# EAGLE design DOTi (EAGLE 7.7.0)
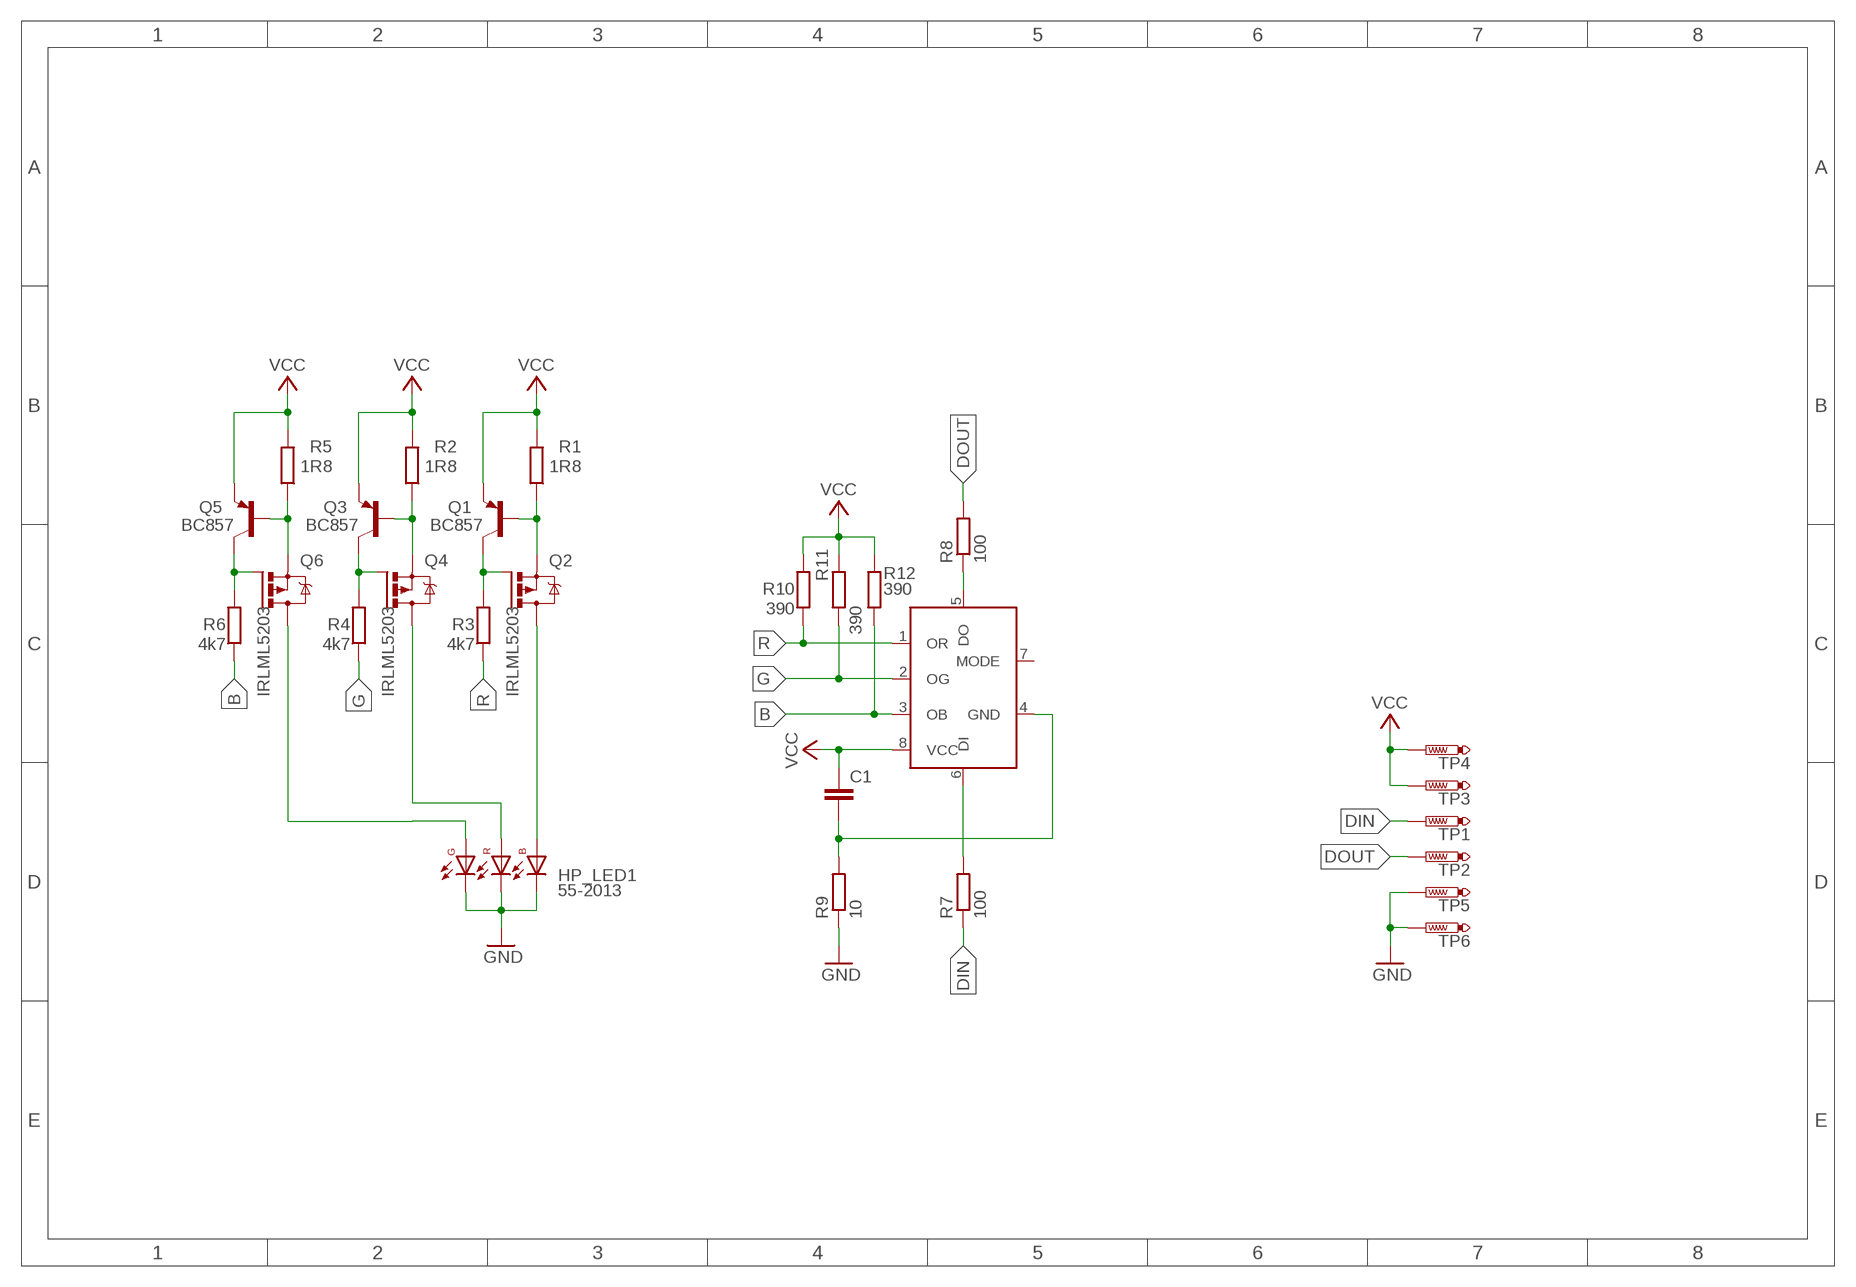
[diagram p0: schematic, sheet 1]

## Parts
C1  C-EUC0603  [C0603]
HP_LED1  55-2013  [HP_RGB_LED]
IC1  WS2811M  [MSOP8]
Q1  BC857  BC857CSMD  [SOT23-BEC]
Q2  IRLML5203  [MICRO3]
Q3  BC857  BC857CSMD  [SOT23-BEC]
Q4  IRLML5203  [MICRO3]
Q5  BC857  BC857CSMD  [SOT23-BEC]
Q6  IRLML5203  [MICRO3]
R1  1R8  R-EU_M1206  [M1206]
R2  1R8  R-EU_M1206  [M1206]
R3  4k7  R-EU_R0603  [R0603]
R4  4k7  R-EU_R0603  [R0603]
R5  1R8  R-EU_M1206  [M1206]
R6  4k7  R-EU_R0603  [R0603]
R7  100  R-EU_R0603  [R0603]
R8  100  R-EU_R0603  [R0603]
R9  10  R-EU_R0603  [R0603]
R10  390  R-EU_R0603  [R0603]
R11  390  R-EU_R0603  [R0603]
R12  390  R-EU_R0603  [R0603]
TP1  PTR1B1,27  [B1,27]
TP2  PTR1B1,27  [B1,27]
TP3  PTR1B1,27  [B1,27]
TP4  PTR1B1,27  [B1,27]
TP5  PTR1B1,27  [B1,27]
TP6  PTR1B1,27  [B1,27]

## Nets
B: IC1.3(OB) R6.1 R12.1
DI: IC1.6(DI) R7.2
DIN: R7.1 TP1.TP
DO: IC1.5(DO) R8.1
DOUT: R8.2 TP2.TP
G: IC1.2(OG) R4.1 R11.1
GND: HP_LED1.1(GC) HP_LED1.2(RC) HP_LED1.3(BC) R9.1 TP5.TP TP6.TP
N$1: HP_LED1.5(RA) Q4.3(D)
N$2: Q1.B Q2.2(S) R1.1
N$3: Q1.C Q2.1(G) R3.2
N$4: HP_LED1.4(BA) Q2.3(D)
N$5: HP_LED1.6(GA) Q6.3(D)
N$6: Q3.B Q4.2(S) R2.1
N$7: Q5.B Q6.2(S) R5.1
N$9: Q3.C Q4.1(G) R4.2
N$11: Q5.C Q6.1(G) R6.2
N$12: C1.2 IC1.4(GND) R9.2
R: IC1.1(OR) R3.1 R10.1
VCC: C1.1 IC1.8(VCC) Q1.E Q3.E Q5.E R1.2 R2.2 R5.2 R10.2 R11.2 R12.2 TP3.TP TP4.TP
Unconnected: IC1.7(MODE)

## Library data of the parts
C1 = rcl:C-EU: CAPACITOR, European symbol
HP_LED1 = RGB_HP_LED:55-2013
IC1 = WS2812:WS2811M
Q1 Q3 Q5 = transistor-pnp:BC857*: PNP Transistror
Q2 Q4 Q6 = transistor-power:IRLML5203: HEXFET P-Channel Power MOSFET
R1-R12 = rcl:R-EU_: RESISTOR, European symbol
TP1-TP6 = testpad:PTR1: TEST PIN

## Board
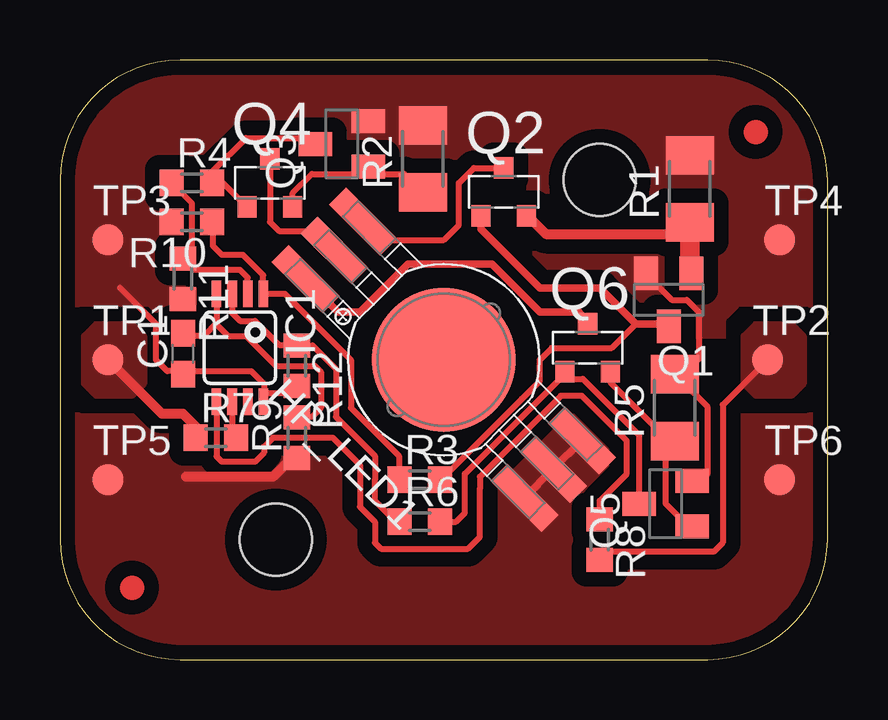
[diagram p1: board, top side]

Size 32 x 25 mm. Coordinates in mm from the lower left corner, seen from the top.
Outline: 5,0 27,0 arc90 32,5 32,20 arc90 27,25 5,25 arc90 0,20 0,5 arc90 5,0
Copper layers (1*16): Top 0.035mm / dielectric 1.5mm / Bottom 0.035mm
Design rules "default *": minimum track width 10mil, minimum drill 24mil, track to track 8mil, track to pad 8mil, pad to pad 8mil, via to via 8mil, smd to smd 8mil, copper to edge 20mil, drill to drill 8mil, minimum pad ring 10mil, minimum via ring 8mil, stop-mask expansion 4mil, vias tented up to drill 0mil, thermal gap 10mil
Holes 3 mm at 9,5 22.5,20

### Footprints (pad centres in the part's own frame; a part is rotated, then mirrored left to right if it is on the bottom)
C0603 = smd 1.1 x 1: 1 -0.85,0; 2 0.85,0
HP_RGB_LED = smd 3 x 1: 1 -6.45,1.7; 2 -6.45,0; 3 -6.45,-1.7; 4 6.45,-1.7; 5 6.45,0; 6 6.45,1.7 | smd 6 x 6: P$1 0,0
MSOP8 = smd 1.1 x 0.4: 1 -2.25,0.975; 2 -2.25,0.325; 3 -2.25,-0.325; 4 -2.25,-0.975; 5 2.25,-0.975; 6 2.25,-0.325; 7 2.25,0.325; 8 2.25,0.975
SOT23-BEC = smd 1 x 1.4: B -0.95,-1.1; C 0,1.1; E 0.95,-1.1
MICRO3 = smd 0.8 x 0.9: 1 -0.95,-1; 2 0.95,-1; 3 0,1
M1206 = smd 1.6 x 2: 1 -1.4,0; 2 1.4,0
R0603 = smd 1 x 1.1: 1 -0.85,0; 2 0.85,0
B1,27 = smd 1.27 x 1.27: TP 0,0

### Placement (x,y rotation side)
C1  5.12,12.75 90 top
HP_LED1  16,12.5 135 top
IC1  7.5,13 270 top
Q1  25.38,15 180 top
Q2  18.5,19.5 0 top
Q3  11.75,21.5 90 top
Q4  8.75,19.88 0 top
Q5  25.25,6.5 90 top
Q6  22,13 0 top
R1  26.25,19.62 90 top
R2  15.12,20.88 90 top
R3  15,7.5 0 top
R4  5.5,19.88 0 top
R5  25.62,10.5 90 top
R6  15,5.75 0 top
R7  6.5,9.25 0 top
R8  22.5,5 270 top
R9  9.88,9.25 90 top
R10  5.5,18.25 180 top
R11  5.12,15.88 270 top
R12  9.88,12.25 270 top
TP1  2,12.5 0 top
TP2  29.5,12.5 0 top
TP3  2,17.5 0 top
TP4  30,17.5 0 top
TP5  2,7.5 0 top
TP6  30,7.5 0 top

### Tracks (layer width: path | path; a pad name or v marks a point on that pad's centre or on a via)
B
  Top 0.254: IC1.3 7.17,14.45 7.5,14.12 8.12,14.12 9.12,13.12 9.85,13.12 R12.1 10.53,13.1 11.25,12.38 11.5,12.12 11.5,10.12 13.12,8.5 13.12,7.5 13.12,6.62 14,5.75
  Top 0.305: R6.1 14,5.75
DI
  Top 0.254: IC1.6 7.17,9.3 R7.2
DIN
  Top 0.254: 2.5,12 TP1.TP
  Top 0.406: R7.1 5.65,9.72 5.12,10.25 4.25,10.25 3.62,10.88 2.5,12
  pour Top (no thermals): 1,11.5 1,13.5 1.5,14 3,14 3.5,13.5 3.5,11.5 3,11 1.5,11
DO
  Top 0.254: R8.1 22.5,6.62 23.62,7.75 23.62,9.12 23.25,9.5 21.75,11 20.88,11 17.5,7.62 17.5,7.12 17.5,5.12 17,4.62 13.38,4.62 13.12,4.88 13.12,5.75 12.5,6.38 12.5,8.12 11.75,8.88 11.38,9.25 8.88,9.25 8.5,8.88 8.5,8.62 8.12,8.25 6.75,8.25 6.53,8.47 IC1.5
DOUT
  Top 0.254: TP2.TP 27.62,10.62 27.62,4.88 27.25,4.5 25.12,4.5 23,4.5 22.52,4 R8.2
  pour Top (isolate 0.406, no thermals): 28.5,13.5 29,14 30.5,14 31,13.5 31,11.5 30.5,11 29,11 28.5,11.5
G
  Top 0.254: IC1.2 7.83,15.93 7.5,16.25 5.6,16.25 R11.1 5.22,16.73 5.5,17 5.5,19.02 R4.1
GND
  Top 0.305: HP_LED1.3 HP_LED1.2 HP_LED1.1 | R9.1 9.65,8.4
  Top 0.406: 9.65,8.4 8.88,7.62 5.25,7.62
  pour Top (isolate 0.61, rank 2, no thermals): 0,11.5 32,11.5 32,0 0,0
N$1
  Top 0.254: Q4.3 8.75,18.25 9.12,17.88 10.62,17.88 HP_LED1.5
N$2
  Top 0.305: 26.25,16.43 Q1.B | Q2.2 19.5,18.5
  Top 0.406: 19.5,18.5 20.25,17.75 25.65,17.75 R1.1
  Top 0.813: R1.1 26.25,16.43
N$3  (1 unrouted)
  Top 0.254: 24,14 23,13 20.5,13 20,12.5 20,11.62 19.25,10.88 15.88,7.5 15.88,7.12
  Top 0.305: 17.55,18.05 Q2.1 17.55,17.95 20,15.5 22.5,15.5 24,14 25.27,14 Q1.C
N$4
  Top 0.254: HP_LED1.4 12.74,18.26 13.5,17.5 16,17.5 16.62,18.12 16.62,19.88 17.25,20.5 Q2.3
N$5
  Top 0.305: HP_LED1.6 11.6,14.5 12,14.5 12.5,14.5 14.5,16.5 16.5,16.5 18,16.5 20,14.5 21.62,14.5 Q6.3
N$6
  Top 0.254: Q4.2 9.7,19.45 10.5,20.25 12.55,20.25 Q3.B 12.95,20.55 13.25,20.25 14.35,20.25 R2.1
N$7
  Top 0.254: Q6.2 22.95,11.55 25.38,9.12 | 25.38,9.12 25.98,9.12 R5.1 | Q5.B 26.2,5.55 25.25,6.5 25.25,9 25.38,9.12
N$9
  Top 0.254: Q4.1 6.8,19.88 R4.2 6.35,20.35 7.75,21.75 10.4,21.75 Q3.C 10.62,21.5 10.25,21.75
N$11
  Top 0.254: Q6.1 21,12 20.88,11.75 16.88,7.75 16.88,6.12 16.5,5.75 R6.2 | 21.05,11.7 21.8,11.7 24.12,9.38 24.12,6.53 Q5.C
  Top 0.305: Q6.1 21.05,11.7
N$12
  Top 0.254: IC1.4 6.53,14.03 | 6.53,14.03 6,13.5 5.22,13.5 C1.2 | 6.53,14.03 6.53,13.97 7,13.5 7.75,13.5 9,12.25 10.62,12.25 10.88,12 10.88,10.5 10.5,10.12 9.9,10.12 R9.2
  Top 0.305: C1.2 5.35,13.6 5.38,13.62 5.12,13.62 C1.2 | C1.2 5.12,13.5
R
  Top 0.254: R3.1 14.12,7.53 14.12,8.5 13.1,9.53 12.12,10.5 12.12,12.5 11.88,12.75 11.75,12.88 9.38,15.25 IC1.1 8.47,16.02 7.62,16.88 6.75,16.88 6.38,17.25 6.38,18.23 R10.1
VCC
  Top 0.254: Q5.E 26.82,7.45 27,7.75 27,10.53 R5.2 26.62,12.53 26.62,14.5 26.12,15 25.5,15 24.43,16.07 Q1.E | 5,12.03 C1.1 | 5,12.03 7.97,12.03 8.5,11.5 | 8.5,11.5 8.5,11.12 | 8.5,11.12 8.5,10.78 IC1.8 | 5,12.03 4.47,12.03 4,12.5 4,14 2.5,15.5 | 8.5,11.5 8.5,11.12 | 8.5,11.12 9.6,11.12 R12.2
  pour Top (isolate 0.61, rank 2, no thermals): 32,13.5 0,13.5 0,25 32,25
(copper drawn outside any net)
  shapes: Top circle x2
